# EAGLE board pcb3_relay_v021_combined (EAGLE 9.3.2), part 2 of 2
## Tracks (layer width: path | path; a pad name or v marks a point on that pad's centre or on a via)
+5V  (via drill 0.35)
  Top 0.61: 21.59,26.04 v21.59,19.43 21.59,10.03 21.08,9.53 IC1.10 | 21.59,26.04 v21.59,36.07 | IC2.16 19.68,33.66 v20.32,34.29 | IC1.16 19.68,17.14 v20.32,17.78 | IC2.10 21.59,26.04
  Top 1.016: C8.1 C30.+ 22.99,72.39 26.42,68.96 v26.42,36.07
  Bottom 0.61: v20.32,34.29 C2.1 | v20.32,17.78 C1.1 17.91,19.05 18.29,19.43 v21.59,19.43
  Bottom 1.016: C8.1 IC4.3 | C2.1 17.91,35.44 18.54,36.07 v21.59,36.07 v26.42,36.07
  other vias: 22.73,72.39
+12V  (via drill 0.35)
  Top 1.016: C15.+ C16.1 22.99,62.36 21.59,60.96 21.59,55.88 22.86,54.61 22.86,30.48 | v27.18,29.46 26.17,30.47 K1.1 22.86,30.48 | v37.34,29.46 36.33,30.47 K2.1 | v47.5,29.46 46.49,30.47 K3.1 | v57.66,29.46 56.65,30.47 K4.1 | v67.82,29.46 66.81,30.47 K5.1 | v77.98,29.46 76.97,30.47 K6.1 | v88.14,29.46 87.13,30.47 K7.1 | v98.3,29.46 97.29,30.47 K8.1 | v108.46,29.46 107.45,30.47 K9.1 | v118.62,29.46 117.61,30.47 K10.1 | v128.78,29.46 127.77,30.47 K11.1 | v138.94,29.46 137.93,30.47 K12.1 | v149.1,29.46 148.09,30.47 K13.1 | v159.26,29.46 158.25,30.47 K14.1 | v169.42,29.46 168.41,30.47 K28.1 | v37.34,10.41 36.33,11.42 K16.1 | K15.1 26.17,11.42 v27.18,10.41 27.18,16 22.86,20.32 22.86,30.48 | v47.5,10.41 46.49,11.42 K17.1 | v57.66,10.41 56.65,11.42 K18.1 | v67.82,10.41 66.81,11.42 K19.1 | v77.98,10.41 76.97,11.42 K20.1 | v88.14,10.41 87.13,11.42 K21.1 | v98.3,10.41 97.29,11.42 K22.1 | v108.46,10.41 107.45,11.42 K23.1 | v118.62,10.41 117.61,11.42 K24.1 | v128.78,10.41 127.77,11.42 K25.1 | v138.94,10.41 137.93,11.42 K26.1 | v149.1,10.41 148.09,11.42 K27.1 | v169.42,10.41 168.41,11.42 K29.1 | IC3.3 v17.78,62.23
  Bottom 1.016: IC4.1 22.86,67.31 24.13,66.04 C16.1 24,62.23 v17.78,62.23 | DS1.C 27.16,29.45 v27.18,29.46 32.89,29.46 33.27,29.08 35.56,29.08 35.94,29.46 v37.34,29.46 | v37.34,29.46 v47.5,29.46 | v47.5,29.46 v57.66,29.46 | v57.66,29.46 v67.82,29.46 | v67.82,29.46 v77.98,29.46 | v77.98,29.46 v88.14,29.46 | v88.14,29.46 v98.3,29.46 | v98.3,29.46 v108.46,29.46 | v108.46,29.46 v118.62,29.46 | v118.62,29.46 v128.78,29.46 | v128.78,29.46 v138.94,29.46 | v138.94,29.46 v149.1,29.46 | v149.1,29.46 v159.26,29.46 | v159.26,29.46 v169.42,29.46 169.4,29.45 DS28.C | DS2.C 37.34,27.96 v37.34,29.46 | DS3.C 47.48,29.45 v47.5,29.46 | DS4.C 57.64,29.45 v57.66,29.46 | DS5.C 67.8,29.45 v67.82,29.46 | DS6.C 77.96,29.45 v77.98,29.46 | DS7.C 88.12,29.45 v88.14,29.46 | DS14.C 159.24,29.45 v159.26,29.46 | DS13.C 149.08,29.45 v149.1,29.46 | DS12.C 138.92,29.45 v138.94,29.46 | DS11.C 128.76,29.45 v128.78,29.46 | DS10.C 118.6,29.45 v118.62,29.46 | DS9.C 108.44,29.45 v108.46,29.46 | DS8.C 98.28,29.45 v98.3,29.46 | v37.34,10.41 v27.18,10.41 27.16,10.4 DS15.C | DS16.C 37.34,8.91 v37.34,10.41 | v37.34,10.41 v47.5,10.41 | DS17.C 47.48,10.4 v47.5,10.41 | v47.5,10.41 v57.66,10.41 | DS18.C 57.66,8.91 v57.66,10.41 | v57.66,10.41 v67.82,10.41 | DS19.C 67.8,10.4 v67.82,10.41 | v67.82,10.41 v77.98,10.41 | DS20.C 77.96,10.4 v77.98,10.41 | v77.98,10.41 v88.14,10.41 | DS21.C 88.14,8.91 v88.14,10.41 | v88.14,10.41 v98.3,10.41 | DS22.C 98.28,10.4 v98.3,10.41 | v98.3,10.41 v108.46,10.41 | DS23.C 108.46,8.91 v108.46,10.41 | v108.46,10.41 v118.62,10.41 | DS24.C 118.6,10.4 v118.62,10.41 | v118.62,10.41 v128.78,10.41 | DS25.C 128.76,10.4 v128.78,10.41 | v128.78,10.41 v138.94,10.41 | DS26.C 138.94,8.91 v138.94,10.41
  Bottom 1.016: v138.94,10.41 v149.1,10.41 | DS27.C 149.08,10.4 v149.1,10.41 | v149.1,10.41 v169.42,10.41 169.42,8.91 DS29.C
  other vias: 24.13,62.36
+15V  (via drill 0.35)
  Top 0.61: IC38.4 158.75,68.45 C38P.1 | IC35.7 153.03,51.44 153.67,52.07 v154.94,52.07 | IC36.7 167,51.44 167.64,52.07 v170.18,52.07 | IC37.7 179.71,51.82 180.21,52.32 182.63,52.32 v182.88,52.07 | IC32.7 126.36,47.62 127,48.26 v128.27,48.26 129.54,49.53 v129.54,52.7 v129.54,58.42 128.27,59.69 v128.27,66.04 | IC31.7 36.2,64.14 36.83,64.77 v38.1,64.77 39.37,63.5 39.37,62.23 38.1,60.96 v38.1,45.72 | IC25.7 52.7,64.64 53.09,65.02 54.48,65.02 54.76,64.75 v54.76,64.64 | IC28.7 52.7,49.15 53.31,49.76 54.51,49.76 v54.68,49.59 v54.67,49.59 | R157.2 R135.2 | IC30.8 97.16,47.88 97.41,48.13 v99.06,48.13 v99.06,58.42 102.87,62.23 v102.87,67.18 101.22,67.18 100.97,66.93 IC27.8 | IC34.7 132.72,68.07 132.97,68.33 134.62,68.33 v134.62,68.2 | v176.53,65.41 E49.TP | IC33.7 122.56,69.09 122.94,69.47 124.84,69.47 v124.97,69.34
  Top 1.016: +15V.TP 5.08,45.72 C66.+ C60.1 | C14.1 C18.+ 16.76,45.72 17.78,46.74 IC3.1 C70.+
  Bottom 0.61: v154.94,52.07 C35P.1 154.94,48.9 | v170.18,52.07 170.56,51.69 C36P.1 170.56,48.9 | v182.88,52.07 C37P.1 182.88,49.53 182.25,48.9 170.56,48.9 | C32P.1 v128.27,48.26 132.08,48.26 132.87,49.05 152.72,49.05 152.88,48.9 154.94,48.9 | v38.1,64.77 C31P.1 C25P.1 54.76,63.52 v54.76,64.64 | v54.67,49.59 54.67,48.19 C28P.1 54.61,45.72 | C14.1 16.26,45.84 16.26,46.61 16.72,47.08 22.77,47.08 24.13,45.72 v38.1,45.72 54.61,45.72 | R157.2 85.26,45.72 84.24,44.7 83.4,44.7 82.38,45.72 54.61,45.72 | v99.06,48.13 C30P.1 | v102.87,67.18 C27P.1 | v134.62,68.2 C34P.1 134.62,65.41 | R135.2 87.63,58.42 v99.06,58.42 v129.54,58.42 | 170.56,48.9 154.94,48.9 | v176.53,65.41 160.02,65.41 | 160.02,65.41 134.62,65.41 | 134.62,65.41 128.91,65.41 v128.27,66.04 125.86,68.45 C33P.1 v124.97,69.34 | R198.1 161.29,76.45 161.8,76.96 176.02,76.96 176.53,77.47 E49.TP | C38P.1 160.02,67.18 160.02,65.41
  Bottom 1.016: C60.1 7.49,46.61 8.38,47.5 12.83,47.5 14.61,45.72 C14.1
  other vias: 159.89,67.31 7.49,45.72 16.38,45.72
-15V  (via drill 0.35)
  Top 0.61: IC31.4 33.66,69.47 33.4,69.72 31.88,69.72 31.75,69.6 C31N.2 v31.75,58.42 | IC25.4 50.16,69.6 49.78,69.98 48.51,69.98 48.26,69.72 C25N.2 v48.26,58.42 48.26,54.48 | IC28.4 50.16,54.48 49.91,54.74 48.51,54.74 48.26,54.48 | 48.26,54.48 C28N.2 | IC30.4 93.34,53.21 93.09,53.47 91.82,53.47 91.44,53.09 | 91.44,53.09 C30N.2 | IC27.4 97.16,72.26 96.9,72.52 v95.25,72.52 | IC32.4 123.83,52.96 123.57,53.21 122.17,53.21 121.92,52.96 C32N.2 v121.92,55.88 | IC33.4 120.02,73.28 119.76,73.53 118.36,73.53 118.11,73.28 C33N.2 v118.11,55.88 | IC34.4 130.18,73.28 129.92,73.53 128.52,73.53 128.27,73.28 C34N.2 | IC35.4 150.5,56.77 150.24,57.02 148.84,57.02 148.59,56.77 C35N.2 | IC36.4 164.47,56.77 164.21,57.02 162.94,57.02 162.56,56.64 | 162.56,56.64 C36N.2 | IC37.4 177.16,57.02 176.91,57.28 175.64,57.28 175.26,56.9 C37N.2 | v162.56,60.96 162.56,56.64 | v158.75,62.1 IC38.11 158.75,66.8 v158.5,67.06 | 91.44,53.09 v91.44,55.88 91.44,69.85 v92.71,71.12 | IC26.14 80.01,57.15 v81.28,55.88 81.28,52.07 80.01,50.8 IC29.14 | v7.62,57.15 7.46,57.3 C71.-
  Top 1.016: -15V.TP 5.08,68.58 C67.- v8.13,68.58 8.13,65.91 7.46,65.25 C71.-
  Bottom 0.61: C37N.2 175,55.75 162.82,55.75 C36N.2 162.56,57.15 162.05,57.66 149.1,57.66 148.59,57.15 C35N.2 122.05,56.01 v121.92,55.88 v118.11,55.88 v91.44,55.88 v81.28,55.88 80.16,57 R152.1 62.08,57.15 60.96,57.15 59.69,58.42 v48.26,58.42 v31.75,58.42 29.21,58.42 27.94,57.15 v7.62,57.15 | R195.1 164.95,60.96 v162.56,60.96 C38N.2 157.61,61.47 158.24,62.1 v158.75,62.1 | v158.5,67.06 158.39,67.16 R196.1 | v95.25,72.52 C27N.2 92.84,71.25 v92.71,71.12
  Bottom 1.016: v8.13,68.58 C61.2 | C33N.2 119.12,73.53 127.89,73.53 128.27,73.15 C34N.2
  other vias: 31.75,68.71 48.26,68.71 48.26,53.47 91.44,52.2 121.92,52.2 118.11,72.52 128.27,72.52 148.59,56.01 162.56,56.01 175.26,56.01
A01  (via drill 0.35)
  Top 0.305: v32.64,21.08 32.71,21.15 K1.5 | v42.8,21.08 42.87,21.15 K2.5 | v52.96,21.08 53.03,21.15 K3.5 | v63.12,21.08 63.19,21.15 K4.5 | v73.28,21.08 73.28,22.8 K5.5 | v83.44,21.08 83.51,21.15 K6.5 | v93.6,21.08 93.67,21.15 K7.5 | v103.76,21.08 103.76,22.8 K8.5 | v113.92,21.08 113.92,22.8 K9.5 | v124.08,21.08 124.08,22.8 K10.5 123.43,22.87 v122.17,24.13
  Bottom 0.305: RA1.1 25.25,21.49 25.65,21.08 v32.64,21.08 v42.8,21.08 v52.96,21.08 v63.12,21.08 v73.28,21.08 v83.44,21.08 v93.6,21.08 v103.76,21.08 v113.92,21.08 v124.08,21.08 | RB11.2 122.3,25.4 | 122.3,25.4 124.46,25.4 125.73,26.67 132.08,26.67 | 132.08,26.67 142.24,26.67 | 142.24,26.67 149.86,26.67 | 149.86,26.67 161.42,26.67 CAC4.2 | CAC3.1 149.73,26.54 149.86,26.67 | CAC2.2 142.37,26.54 142.24,26.67 | CAC1.2 132.21,26.54 132.08,26.67 | v122.17,24.13 122.17,25.27 122.3,25.4
A02  (via drill 0.35)
  Top 0.305: v25.65,1.65 25.71,1.71 K15.4 | v35.81,1.65 35.87,1.71 K16.4 | v45.97,1.65 46.03,1.71 K17.4 | v56.13,1.65 56.19,1.71 K18.4 | v66.29,1.65 66.35,1.71 K19.4 | v76.45,1.65 76.51,1.71 K20.4 | v86.61,1.65 86.67,1.71 K21.4 | v96.9,1.65 96.9,3.75 K22.4 | v106.93,1.65 106.99,1.71 K23.4 | v117.09,1.65 117.15,1.71 K24.4 | v127.25,1.65 127.31,1.71 K25.4 | v137.41,1.65 137.47,1.71 K26.4 v140.96,3.82 v140.97,3.81 | v147.57,1.65 147.63,1.71 K27.4 v151.12,3.82 v151.13,3.81 | v157.99,1.65 157.99,3.62 157.8,3.81 v156.21,3.81
  Bottom 0.305: v157.99,1.65 v147.58,1.65 v147.57,1.65 v137.41,1.65 v127.25,1.65 v117.09,1.65 v106.93,1.65 v96.9,1.65 v86.61,1.65 v76.45,1.65 v66.29,1.65 v56.13,1.65 v45.97,1.65 v35.82,1.65 v35.81,1.65 v25.65,1.65 23.75,1.65 22.86,2.54 RC1.1 | v140.97,3.81 CDF1.2 | CDF3.1 v156.21,3.81 | v151.13,3.81 CDF2.2
ACONT  (via drill 0.35)
  Top 0.305: IC27.1 100.97,72.26 v101.35,72.64 | C55.- v107.95,73.77 107.95,74.93 106.68,76.2 E23.TP | v87.63,73.66 87.63,77.47 CON1.8
  Bottom 0.305: v107.95,73.77 106.36,73.77 D16.2 104.73,72.64 v101.35,72.64 98.81,72.64 97.79,73.66 v87.63,73.66
AD_DIST  (via drill 0.35)
  Top 0.254: v116.84,78.74 v116.84,40.01
  Top 0.305: CON2.2 2.54,25.4 1.27,26.67 1.27,38.73 v2.54,40.01 | v179.07,46.99 177.67,45.59 v177.67,40.01
  Bottom 0.254: E42.TP v116.84,78.74
  Bottom 0.305: v177.67,40.01 v116.84,40.01 v2.54,40.01 | R1.2 v179.07,46.99 R193.1
E21  (via drill 0.35)
  Top 0.305: v43.18,46.99 E21.TP
  Bottom 0.305: R145.2 50.95,46.99 v43.18,46.99 | E21.TP 52.07,80.01 53.85,78.23 77.47,78.23 79.25,80.01 82.55,80.01 CON1.4
E29  (via drill 0.35)
  Top 0.305: E29.TP 30.48,39.37 29.21,38.1 v29.21,20.32 | v25.4,20.32 25.4,22.56 K1.4 | K2.4 35.56,22.56 v35.56,20.32 | v45.72,20.32 45.72,22.56 K3.4 | v55.88,20.32 55.88,22.56 K4.4 | v66.04,20.32 66.04,22.56 K5.4 | v76.2,20.32 76.2,22.56 K6.4 | v86.36,20.32 86.36,22.56 K7.4 | v96.52,20.32 96.52,22.56 K8.4 | v106.68,20.32 106.68,22.56 K9.4 | v116.84,20.32 116.84,22.56 K10.4 | R167.1 v35.56,78.74
  Bottom 0.305: v116.84,20.32 v106.68,20.32 v96.52,20.32 v86.36,20.32 v76.2,20.32 v66.04,20.32 v55.88,20.32 v45.72,20.32 v35.56,20.32 v29.21,20.32 v25.4,20.32 23.62,20.32 22.86,21.08 RB1.1 | E29.TP 31.75,78.74 v35.56,78.74 41.63,78.74 41.65,78.72 44.71,78.72 44.73,78.74 50.8,78.74 52.07,77.47 81.66,77.47 82.93,76.2 CON1.3
E31  (via drill 0.35)
  Top 0.305: IC38.2 v161.29,73.66 | v157.48,73.66 IC38.5 | E31.TP v113.03,76.2
  Bottom 0.305: v161.29,73.66 v157.48,73.66 143.51,73.66 140.97,76.2 v113.03,76.2 95.25,76.2 93.98,77.47 82.55,77.47 CON1.2
E32  (via drill 0.35)
  Top 0.305: C52.+ 69.85,71.63 73.66,75.44 v73.66,76.2 v73.66,80.01
  Bottom 0.305: E32.TP v73.66,80.01 | CON1.1 v73.66,76.2
E34  (via drill 0.35)
  Top 0.305: v129.67,20.95 v129.67,45.21
  Bottom 0.305: 150.11,20.95 157.35,20.95 | 157.35,20.95 166.62,20.95 | 166.62,20.95 170.81,20.95 171.32,21.46 171.32,22.84 R171.2 | CEG4.2 166.5,21.08 166.62,20.95 | CEG2.2 149.99,21.08 150.11,20.95 | CEG3.1 157.35,20.96 157.35,20.95 | 139.83,20.95 v129.67,20.95 129.69,20.98 RA11.2 | 139.83,20.95 150.11,20.95 | CEG1.2 139.83,20.96 139.83,20.95 | v129.67,45.21 126.36,45.21 125.73,45.85 R172.1
E35  (via drill 0.35)
  Top 0.305: K11.4 127.31,21.28 v128.27,20.32 | v137.16,20.32 137.47,20.63 K12.4 | v147.32,20.32 147.63,20.63 K13.4 | v157.48,20.32 157.79,20.63 K14.4 | v149.86,7.56 149.99,7.69 v149.99,20.32 | v130.81,20.32 130.81,27.43 130.69,27.55 v130.69,45.34 v130.68,45.34
  Bottom 0.305: 142.24,7.56 137.86,7.56 137.8,7.62 133.48,7.62 CBD1.2 | 142.24,7.56 v149.86,7.56 149.86,6.48 CBD3.1 | CBD2.2 142.24,6.48 142.24,7.56 | v128.27,20.32 v130.81,20.32 v137.16,20.32 v147.32,20.32 v149.99,20.32 v157.48,20.32 | R173.2 130.68,46.71 v130.68,45.34
E36  (via drill 0.35)
  Top 0.305: v32.64,2.29 32.71,2.36 K15.5 | v42.8,2.29 42.87,2.36 K16.5 | v52.96,2.29 53.03,2.36 K17.5 | v63.12,2.29 63.19,2.36 K18.5 | v73.28,2.29 73.35,2.36 K19.5 | v83.44,2.29 83.51,2.36 K20.5 | v93.6,2.29 93.67,2.36 K21.5 | v103.76,2.29 103.83,2.36 K22.5 | v113.92,2.29 113.99,2.36 K23.5 | v124.08,2.29 124.15,2.36 K24.5 | v134.24,2.29 134.31,2.36 K25.5 | v144.4,2.29 144.47,2.36 K26.5 | v154.56,2.29 154.63,2.36 K27.5 | v119.13,67.94 119.13,65.41 119.51,65.02 v119.51,2.29
  Bottom 0.305: RD1.1 25.25,2.56 25.53,2.29 v32.64,2.29 v42.8,2.29 v52.96,2.29 v63.12,2.29 v73.28,2.29 v83.44,2.29 v93.6,2.29 v103.76,2.29 v113.92,2.29 v119.51,2.29 v124.08,2.29 v134.24,2.29 v144.4,2.29 v154.56,2.29 | v119.13,67.94 119.61,68.43 R175.1 R174.2
E38  (via drill 0.35)
  Top 0.305: v125.73,6.35 125.73,13.46 125.48,13.71 125.48,35.82 125.73,36.08 125.73,64.52 v125.86,64.64
  Bottom 0.305: RC11.2 v125.73,6.35 | R207.1 v125.86,64.64
E40  (via drill 0.35)
  Top 0.305: v137.16,50.8 137.16,59.69 135.89,60.96 R180.1 v135.89,78.74 | IC34.6 v131.44,63.5 v131.45,63.5
  Bottom 0.305: R182.1 152.25,50.8 v137.16,50.8 | v135.89,78.74 E40.TP | R180.1 134.62,63.5 v131.45,63.5
E43
  Bottom 0.305: R200.2 E43.TP
E44
  Bottom 0.305: E44.TP 151.13,77.47 R201.2
E45
  Bottom 0.305: R202.2 E45.TP
E46  (via drill 0.35)
  Top 0.305: v166.37,76.18 166.37,77.47 E46.TP
  Bottom 0.305: R203.2 v166.37,76.18
FCONT  (via drill 0.35)
  Top 0.305: IC38.9 v156.21,62.99 | v160.02,62.99 IC38.12 | IC30.1 v97.16,53.72 | C59.- v104.14,53.72 107.95,57.53 v107.95,61.59 107.95,62.23 105.41,64.77 v105.41,75.05 | v100.33,74.93 E22.TP
  Bottom 0.305: v160.02,62.99 v156.21,62.99 154.43,62.99 153.67,62.23 138.43,62.23 137.16,60.96 120.65,60.96 120.02,61.59 v107.95,61.59 | v97.16,53.72 v104.14,53.72 109.81,53.72 D21.2 | v105.41,75.05 100.45,75.05 v100.33,74.93 92.71,74.93 91.44,76.2 CON1.7
GND  (via drill 0.35)
  Top 0.305: K28.3 169.37,25.07 v169.42,25.02 | IC34.3 v131.44,73.91
  Bottom 0.305: RD11.2 v132.08,3.81 | R199.1 v163.83,76.18 | C36P.2 v170.56,54.74
  pour Top (isolate 0.406): 0,82.55 189.23,82.55 189.23,0 0,0
  pour Bottom (isolate 0.305): 0,82.55 189.23,82.55 189.23,0 0,0
N$1  (via drill 0.35)
  Top 0.305: v70.87,66.02 70.87,65.02 72.39,63.5 IC26.8
  Bottom 0.305: v70.87,66.02 70.98,66.14 R130.1
N$2  (via drill 0.35)
  Top 0.305: R192.1 v184.15,45.72
  Bottom 0.305: v184.15,45.72 184.15,46.84 R193.2
N$3  (via drill 0.35)
  Top 0.305: IC37.3 v178.44,57.53
  Bottom 0.305: v178.44,57.53 180.09,57.53 180.34,57.28 R190.2
N$4  (via drill 0.35)
  Top 0.305: IC36.2 167,55.24 v167.64,54.61
  Bottom 0.305: v167.64,54.61 R186.1 R187.2 164.41,53.49 163.59,54.31 160.51,54.31 R185.1
N$5  (via drill 0.35)
  Top 0.305: v167,43.81 167,44.83 165.1,46.73 v165.1,52.07
  Bottom 0.305: D23.1 v167,43.81 | v165.1,52.07 R187.1
N$6  (via drill 0.35)
  Top 0.305: IC36.6 v165.74,46.99 | v162.56,43.81 v162.56,46.99
  Bottom 0.305: v165.74,46.99 D22.1 v162.56,46.99 | D23.2 v162.56,43.81
N$7  (via drill 0.35)
  Top 0.305: v172.72,49.68 v172.72,46.99 | v169.06,50.8 169.06,47.01 v169.04,46.99
  Bottom 0.305: R188.1 v172.72,49.68 | v172.72,46.99 v169.04,46.99 D22.2 | R186.2 167.79,50.8 v169.06,50.8
N$8  (via drill 0.35)
  Top 0.305: v172.72,54.61 v172.72,58.42 | v179.71,58.42 IC37.2 | C74.- v185.42,58.42
  Bottom 0.305: R188.2 v172.72,54.61 | R189.1 172.87,58.27 v172.72,58.42 177.8,58.42 | v185.42,58.42 v179.71,58.42 177.8,58.42 | R191.1 177.8,57.15 177.8,57.53 177.8,58.42
N$9  (via drill 0.35)
  Top 0.305: v177.86,52.13 178.44,51.55 IC37.6 178.44,48.9 180.34,46.99 180.34,43.18 | 180.34,43.18 R192.3 | 180.34,43.18 R192.2 | C74.+ v185.42,44.45
  Bottom 0.305: v177.86,52.13 177.8,52.18 R191.2 | v185.42,44.45 182.88,44.45 R192.2
N$10  (via drill 0.35)
  Top 0.305: C73.- 160.02,57.15 | 160.02,57.15 v160.02,58.44 | v158.75,56.87 159.03,57.15 160.02,57.15
  Bottom 0.305: v160.02,58.44 160.04,58.42 168.76,58.42 R189.2 | R185.2 159.38,56.24 v158.75,56.87
N$11  (via drill 0.35)
  Top 0.305: IC38.13 v161.29,63.12
  Bottom 0.305: R194.2 R195.2 163.98,63.65 163.45,63.12 v161.29,63.12
N$12  (via drill 0.35)
  Top 0.305: IC38.3 160.02,72.26 v160.15,72.39
  Bottom 0.305: v160.15,72.39 161.14,72.39 R198.2 R199.2
N$13  (via drill 0.35)
  Top 0.305: v156.21,71.12 IC38.6
  Bottom 0.305: R196.2 v156.21,71.12 154.79,71.12 R197.2
N$14  (via drill 0.35)
  Top 0.305: IC38.1 v162.56,73.66
  Bottom 0.305: R203.1 166.37,73.28 165.99,73.66 v162.56,73.66
N$15  (via drill 0.35)
  Top 0.305: v171.45,76.18 E47.TP
  Bottom 0.305: R204.2 v171.45,76.18
N$16  (via drill 0.35)
  Top 0.305: IC35.2 153.03,59.05 v152.4,59.69
  Bottom 0.305: R183.1 R184.2 v152.4,59.69
N$17  (via drill 0.35)
  Top 0.305: IC25.2 52.7,70.48 50.95,72.24 R127.1 v50.8,73.66
  Bottom 0.305: R125.1 v50.8,73.66
N$18  (via drill 0.35)
  Top 0.305: IC38.7 154.94,71.88 v155.19,72.14
  Bottom 0.305: v155.19,72.14 155.3,72.24 R202.1
N$19  (via drill 0.35)
  Top 0.305: v153.67,69.85 153.67,68.58 154.94,67.31 IC38.8
  Bottom 0.305: v153.67,69.85 152.4,69.85 151.13,71.12 R201.1
N$20  (via drill 0.35)
  Top 0.305: v25.65,26.04 25.71,25.98 K1.3
  Bottom 0.305: RB2.1 27.64,25.55 25.65,25.55 | 25.65,25.55 RB1.2 | v25.65,26.04 25.65,25.55
N$21
  Top 0.305: R179.2 136.04,58.9 133.35,61.59 R180.2
  Bottom 0.305: R180.3 R180.2
N$22
  Top 0.305: R127.2 R126.1 55.6,75.08 D12.1 D13.2
N$23  (via drill 0.35)
  Top 0.305: v35.31,26.04 35.31,25.65 35.87,25.09 K2.3
  Bottom 0.305: RB2.2 31.27,26.04 v35.31,26.04 37.31,26.04 RB3.1
N$24  (via drill 0.35)
  Top 0.305: D13.1 D12.2 | D12.2 55.6,72.24 R126.2 | IC25.6 51.44,65.41 v52.07,66.04 | C53.+ 58.31,65.07 v58.31,67.31 58.31,69.53 D12.2
  Bottom 0.305: v52.07,66.04 53.34,67.31 v58.31,67.31
N$25  (via drill 0.35)
  Top 0.305: v163.83,68.58 162.56,67.31 IC38.14 | v146.05,68.58 v146.05,71.12
  Bottom 0.305: v146.05,71.12 R200.1 | v163.83,68.58 v146.05,68.58
N$26  (via drill 0.35)
  Top 0.305: v45.47,26.16 45.47,25.63 K3.3
  Bottom 0.305: RB3.2 41.55,26.16 v45.47,26.16 47.35,26.16 RB4.1
N$27  (via drill 0.35)
  Top 0.305: v53.34,57 52.7,56.36 IC28.2 52.7,52.32 v52.07,51.69
  Bottom 0.305: R146.1 v53.34,57 54.33,57 D17.1 D18.2 | v52.07,51.69 R145.1
N$28  (via drill 0.35)
  Top 0.305: C56.- 58.61,53.34 v59.69,53.34
  Bottom 0.305: v59.69,53.34 58.57,52.22 | 58.57,52.22 R147.1 | R148.2 62.23,49.53 59.54,52.22 58.57,52.22
N$29  (via drill 0.35)
  Top 0.305: IC28.6 51.44,45.09 v52.07,44.45 | v58.42,44.45 C56.+ 58.42,49.53 56.52,51.44 v56.52,60.12
  Bottom 0.305: D18.1 v56.52,60.12 D17.2 52.35,60.12 R146.2 | v52.07,44.45 v58.42,44.45
N$30  (via drill 0.35)
  Top 0.305: IC26.3 v77.47,64.77
  Bottom 0.305: v77.47,64.77 77.32,64.62 R137.2
N$31  (via drill 0.35)
  Top 0.305: v81.28,69.34 81.28,67.42 81.39,67.31 81.39,66.79 81.28,66.68 v81.28,58.4 | IC26.10 v74.93,59.69
  Bottom 0.305: R129.1 v81.28,69.34 | v81.28,58.4 81.26,58.42 81.26,58.44 80.01,59.69 v74.93,59.69
N$32  (via drill 0.35)
  Top 0.305: K4.3 55.86,25.4 55.86,26.05 v55.75,26.16
  Bottom 0.305: RB4.2 51.71,26.16 v55.75,26.16 57.51,26.16 RB5.1
N$33  (via drill 0.35)
  Top 0.305: IC32.6 v125.09,44.45 v125.1,44.45 | v131.44,44.45 v131.44,50.93 v131.44,55.12 | IC32.2 v126.36,55.12
  Bottom 0.305: v125.1,44.45 v131.44,44.45 | v126.36,55.12 v131.44,55.12 | R173.1 130.56,50.04 v131.44,50.93
N$34  (via drill 0.35)
  Top 0.305: IC32.3 125.09,50.42 v124.33,49.66
  Bottom 0.305: v124.33,49.66 124.36,49.68 R172.2
N$35  (via drill 0.35)
  Top 0.305: IC29.2 v78.74,53.34
  Bottom 0.305: v78.74,53.34 78.74,52.22 R159.1
N$36  (via drill 0.35)
  Top 0.305: v82.55,59.69 82.55,58.42 R135.3
  Bottom 0.305: R134.1 v82.55,59.69
N$37  (via drill 0.35)
  Top 0.305: IC26.2 v78.74,63.5
  Bottom 0.305: v78.74,63.5 R137.1
N$38  (via drill 0.35)
  Top 0.305: IC26.5 v74.93,72.64 | v83.82,72.64 v83.82,66.04
  Bottom 0.305: v83.82,72.64 v74.93,72.64 | v83.82,66.04 78.89,66.04 R133.1
N$39  (via drill 0.35)
  Top 0.305: IC29.5 74.93,53.59 v74.42,53.09
  Bottom 0.305: v74.42,53.09 73.81,53.7 R155.1
N$40  (via drill 0.35)
  Top 0.305: IC29.8 72.39,50.8 v71.12,52.07
  Bottom 0.305: v71.12,52.07 R154.1
N$41  (via drill 0.35)
  Top 0.305: v76.2,74.91 IC26.4 | v67.31,74.93 v67.31,71.12
  Bottom 0.305: v67.31,71.12 R131.1 | v76.2,74.91 67.33,74.91 v67.31,74.93
N$42  (via drill 0.35)
  Top 0.305: IC26.1 80.76,66.95 v80.76,67.05
  Bottom 0.305: v80.76,67.05 77.47,67.05 77.06,67.46 R132.1
N$43  (via drill 0.35)
  Top 0.305: C52.- v69.85,73.91
  Bottom 0.305: R129.2 R128.1 78.64,73.91 v69.85,73.91
N$44  (via drill 0.35)
  Top 0.305: IC29.12 77.47,44.29 v78.74,43.02 | v85.09,52.07 v85.09,44.45
  Bottom 0.305: v78.74,43.02 78.9,43.18 80.14,43.18 C58.1 81.51,44.09 84.49,44.09 84.85,44.45 v85.09,44.45 | R156.2 84.94,52.22 v85.09,52.07 86.21,52.07 R160.2
N$45  (via drill 0.35)
  Top 0.305: v73.28,63.5 73.66,63.88 IC26.6 v73.66,68.58 | v85.09,64.77 v85.09,67.31
  Bottom 0.305: R139.1 72.26,62.21 C54.2 v73.28,63.5 | R136.1 v85.09,64.77 | v73.66,68.58 76.71,68.58 77.72,67.56 80.01,67.56 80.39,67.94 84.45,67.94 v85.09,67.31
N$46  (via drill 0.35)
  Top 0.305: IC26.12 77.47,62.02 v77.57,62.12
  Bottom 0.305: R138.2 87.63,63.5 86.36,62.23 82.55,62.23 | C54.1 76.39,62.17 77.28,62.17 77.33,62.12 v77.57,62.12 77.69,62.23 82.55,62.23 | R134.2 82.55,62.23
N$47  (via drill 0.35)
  Top 0.305: v96.65,68.58 97.16,68.07 IC27.5 97.16,59.84 v96.52,59.2
  Bottom 0.305: v96.65,68.58 R140.1 | v96.52,59.2 96.34,59.03 81.94,59.03 80.01,60.96 R139.2
N$48  (via drill 0.35)
  Top 0.305: IC27.6 98.42,64.77 v97.92,64.26
  Bottom 0.305: v97.92,64.26 97.79,64.14 R141.2 91.59,63.65 88.75,60.81 R138.1
N$49  (via drill 0.35)
  Top 0.305: IC29.10 v74.93,47.88
  Bottom 0.305: v74.93,47.88 74.93,48.41 R148.1
N$50  (via drill 0.35)
  Top 0.305: IC27.7 v99.69,60.81
  Bottom 0.305: D15.2 D14.1 102.39,60.02 R142.2 v99.69,60.81 R141.1
N$51
  Bottom 0.305: D15.1 D14.2 | D14.2 R143.2 | D14.2 101.83,63.42 R142.1
N$52  (via drill 0.35)
  Top 0.305: IC27.2 99.69,73.03 v100.33,73.66
  Bottom 0.305: R143.1 R144.2 108.38,69.16 D16.1 108.84,72.85 108.84,74.04 108.46,74.42 101.09,74.42 v100.33,73.66
N$53  (via drill 0.35)
  Top 0.305: v107.95,64.77 C55.+
  Bottom 0.305: R144.1 v107.95,64.77
N$54  (via drill 0.35)
  Top 0.305: v59.69,71.12 C53.- 60.77,67.31 v60.96,67.31
  Bottom 0.305: v59.69,71.12 R131.2 | R150.2 62.08,67.31 v60.96,67.31 59.84,67.31 R153.1
N$55  (via drill 0.35)
  Top 0.305: R135.1 88.9,58.42 87.63,59.69 v85.09,59.69
  Bottom 0.305: v85.09,59.69 R136.2
N$56  (via drill 0.35)
  Top 0.305: v60.96,58.42 v60.96,63.5 | IC29.4 76.2,57.76 v76.22,57.78
  Bottom 0.305: v60.96,58.42 63.5,58.42 64.14,57.78 v76.22,57.78 | v60.96,63.5 59.84,64.62 R153.2
N$57  (via drill 0.35)
  Top 0.305: IC29.3 v77.47,52.07
  Bottom 0.305: v77.47,52.07 R159.2
N$58
  Bottom 0.305: R157.3 R156.1
N$59  (via drill 0.35)
  Top 0.305: v88.9,50.8 R157.1
  Bottom 0.305: R158.2 82.7,50.8 v88.9,50.8
N$60  (via drill 0.35)
  Top 0.305: IC29.6 73.66,52.96 73.03,52.33 73.03,47.76 73.03,47.75 v73.03,47.12
  Bottom 0.305: R158.1 C58.2 81.26,47.14 R161.1 78.72,47.12 v73.03,47.12
N$61  (via drill 0.35)
  Top 0.305: v92.71,43.18 93.34,43.81 IC30.5 93.34,49.01 v92.82,49.53
  Bottom 0.305: v92.71,43.18 80.79,43.18 79.99,42.39 78.48,42.39 78.11,42.76 78.11,43.28 78.74,43.91 R161.2 | v92.82,49.53 R162.1
N$62  (via drill 0.35)
  Top 0.305: IC30.6 94.61,45.96 v94.49,45.83 | v90.04,49.4 v90.04,44.45
  Bottom 0.305: v94.49,45.83 91.93,45.83 91.29,45.19 R163.2 v90.04,44.45 | R160.1 90.02,49.38 v90.04,49.4
N$63
  Bottom 0.305: R165.1 101.6,44.45 102.87,45.72 D19.1 D20.2 106.96,46.84 R164.2
N$64  (via drill 0.35)
  Top 0.305: IC30.2 95.89,53.98 v96.52,54.61 | v107.95,54.61 v107.95,49.96 | v111.76,49.66 111.76,53.59 v112.14,53.98
  Bottom 0.305: D19.2 D20.1 v107.95,49.96 110.21,49.96 R164.1 111.78,49.68 | v96.52,54.61 v107.95,54.61 | R166.2 111.78,49.68 | 111.78,49.68 v111.76,49.66 | v112.14,53.98 D21.1
N$65  (via drill 0.35)
  Top 0.305: IC31.6 34.92,66.67 34.29,67.31 v34.29,77.47 | v45.72,77.47 C72.- | R170.1 v40.64,77.47
  Bottom 0.305: v34.29,77.47 v40.64,77.47 v45.72,77.47
N$66  (via drill 0.35)
  Top 0.305: v104.14,44.45 C59.+
  Bottom 0.305: R166.1 113.03,45.72 111.76,44.45 v104.14,44.45
N$67  (via drill 0.35)
  Top 0.305: IC29.1 80.01,55.96 v79.76,56.21
  Bottom 0.305: v79.76,56.21 67.9,56.21 67.46,55.78 R2.2
N$68  (via drill 0.35)
  Top 0.305: v64.64,63.37 v64.64,55.97
  Bottom 0.305: v64.64,63.37 64.64,64.49 R149.2 R132.2 | R2.1 64.62,55.95 v64.64,55.97
N$69  (via drill 0.35)
  Top 0.305: v67.31,69.85 C57.- | v63.5,59.69 v63.5,66.04
  Bottom 0.305: R149.1 64.92,67.46 | 64.92,67.46 v67.31,69.85 | R151.2 v63.5,59.69 63.35,59.84 R152.2 | 64.92,67.46 v63.5,66.04 62.23,64.77 R150.1
N$70  (via drill 0.35)
  Top 0.305: IC30.7 95.89,45.09 v95.25,44.45
  Bottom 0.305: R163.1 v95.25,44.45 R165.2
N$71
  Top 0.305: IC31.3 34.92,70.48 35.56,71.12 R167.2
N$72  (via drill 0.35)
  Top 0.305: R169.2 v40.64,40.64 | K28.4 166.74,22.87 166.45,23.16 166.45,34.24 167.13,34.92 v167.13,40.64
  Bottom 0.305: v40.64,40.64 165.87,40.64 v167.13,40.64
N$73
  Top 0.305: IC31.2 36.2,69.85 37.47,71.12 40.64,71.12 | R169.1 40.64,71.12 | 40.64,71.12 R170.2
N$74  (via drill 0.35)
  Top 0.305: v158.37,14.22 v158.37,9.14
  Bottom 0.305: D2.1 158.32,14.18 | 158.32,14.18 v158.37,14.22 | v158.37,9.14 158.62,8.89 RS31.1 | RS27.2 155.28,14.18 158.32,14.18 | D1.1 158.32,14.18
N$75  (via drill 0.35)
  Top 0.305: v120.65,69.85 121.28,70.48 IC33.3
  Bottom 0.305: R175.2 v120.65,69.85
N$76  (via drill 0.35)
  Top 0.305: v121.28,63.25 IC33.6 121.28,69.22 122.56,70.48 IC33.2
  Bottom 0.305: R176.1 122.3,62.23 v121.28,63.25 121.89,63.86 R207.2
N$79  (via drill 0.35)
  Top 0.305: v169.16,5.97 169.11,6.02 K29.3 166.7,6.02 166.37,6.35 166.37,10.54 165.74,11.17 v165.74,20.32 | v161.29,46.99 161.29,29.98 161.24,29.93 161.24,27.6 161.29,27.55 v161.29,20.32 | v133.35,60.33 134.62,59.05 v134.62,46.99 | v129.54,60.33 v129.54,62.23
  Bottom 0.305: R177.1 169.7,6.5 v169.16,5.97 | v165.74,20.32 v161.29,20.32 | v134.62,46.99 v161.29,46.99 | v133.35,60.33 v129.54,60.33 | v129.54,62.23 R176.2
N$80  (via drill 0.35)
  Top 0.305: K29.4 169.03,3.82 v169.16,3.68 170.31,4.83 170.31,44.7 v169.29,45.72 | IC34.2 132.72,70.23 132.08,69.6 132.08,55.88 | v132.08,45.72 132.08,55.88 | R179.1 132.08,55.88
  Bottom 0.305: v169.16,3.68 169.19,3.66 R177.2 | v169.29,45.72 v132.08,45.72
N$81  (via drill 0.35)
  Top 0.305: v152.4,54.61 151.76,55.24 IC35.3
  Bottom 0.305: R182.2 v152.4,54.61
N$84  (via drill 0.35)
  Top 0.305: v152.4,48.26 151.76,48.9 IC35.6 151.76,52.7 151.13,53.34 151.13,63.5 v151.26,63.63 | v160.02,48.11 C73.+
  Bottom 0.305: v152.4,48.26 159.87,48.26 v160.02,48.11 | R184.1 151.28,63.65 v151.26,63.63
N$85  (via drill 0.35)
  Top 0.305: v65.91,26.16 65.91,25.51 K5.3
  Bottom 0.305: RB5.2 61.87,26.16 v65.91,26.16 67.67,26.16 RB6.1
N$86  (via drill 0.35)
  Top 0.305: K6.3 76.18,25.4 76.18,25.93 v75.95,26.16
  Bottom 0.305: RB6.2 72.03,26.16 v75.95,26.16 77.83,26.16 RB7.1
N$87  (via drill 0.35)
  Top 0.305: v86.11,26.16 86.11,25.63 K7.3
  Bottom 0.305: RB7.2 82.19,26.16 v86.11,26.16 87.99,26.16 RB8.1
N$88  (via drill 0.35)
  Top 0.305: K8.3 96.5,25.4 96.5,26.05 v96.39,26.16
  Bottom 0.305: RB8.2 92.35,26.16 v96.39,26.16 98.15,26.16 RB9.1
N$89  (via drill 0.35)
  Top 0.305: v106.55,26.16 106.55,25.51 K9.3
  Bottom 0.305: RB9.2 102.51,26.16 v106.55,26.16 108.31,26.16 RB10.1
N$90  (via drill 0.35)
  Top 0.305: v116.59,26.16 116.59,25.63 K10.3
  Bottom 0.305: RB10.2 112.67,26.16 v116.59,26.16 118.47,26.16 RB11.1
N$91  (via drill 0.35)
  Top 0.305: v33.27,24 32.71,24.57 K1.6
  Bottom 0.305: RA1.2 29.23,24 v33.27,24 34.27,24 RA2.1
N$92  (via drill 0.35)
  Top 0.305: K2.6 42.87,25.09 43.43,24.53 v43.43,24
  Bottom 0.305: RA2.2 39.4,24 v43.43,24 44.42,24 RA3.1
N$93  (via drill 0.35)
  Top 0.305: K3.6 53.59,24.51 v53.59,24
  Bottom 0.305: RA3.2 49.55,24 v53.59,24 54.59,24 RA4.1
N$94  (via drill 0.35)
  Top 0.305: K4.6 63.5,24.76 v63.5,24
  Bottom 0.305: RA4.2 59.72,24 v63.5,24 64.75,24 RA5.1
N$95  (via drill 0.35)
  Top 0.305: v73.66,24.13 73.66,25.4 73.35,25.09 K5.6
  Bottom 0.305: RA5.2 70,24.13 v73.66,24.13 74.78,24.13 RA6.1
N$96  (via drill 0.35)
  Top 0.305: v83.82,24.13 83.82,25.4 83.51,25.09 K6.6
  Bottom 0.305: RA6.2 80.16,24.13 v83.82,24.13 84.94,24.13 RA7.1
N$97  (via drill 0.35)
  Top 0.305: v93.98,24.13 93.98,25.4 93.67,25.09 K7.6
  Bottom 0.305: RA7.2 90.32,24.13 v93.98,24.13 95.1,24.13 RA8.1
N$98  (via drill 0.35)
  Top 0.305: v104.14,24.13 104.14,25.4 103.83,25.09 K8.6
  Bottom 0.305: RA8.2 100.48,24.13 v104.14,24.13 105.26,24.13 RA9.1
N$99  (via drill 0.35)
  Top 0.305: K9.6 114.68,24.38 v114.68,24
  Bottom 0.305: RA9.2 110.52,24 v114.68,24 115.55,24 RA10.1
N$100  (via drill 0.35)
  Top 0.305: K10.6 123.83,24.75 v123.83,23.96
  Bottom 0.305: RA11.1 125.74,23.96 v123.83,23.96 123.41,23.96 122.3,22.86 RA10.2
N$101  (via drill 0.35)
  Top 0.305: v29.84,34.16 30.14,34.46 QS1.1
  Bottom 0.305: RS1.1 30.35,34.67 v29.84,34.16
N$102  (via drill 0.35)
  Top 0.508: QS1.3 31.75,30.6 31.62,30.47
  Top 1.016: v30.1,27.94 30.1,29.46 31.11,30.48 31.12,30.47 31.62,30.47 K1.8
  Bottom 1.016: DS1.A v30.1,27.94
N$103  (via drill 0.35)
  Top 0.305: v40.01,34.16 40.3,34.46 QS2.1
  Bottom 0.305: RS2.1 40.51,34.67 v40.01,34.16
N$104  (via drill 0.35)
  Top 0.508: QS2.3 41.91,30.47
  Top 1.016: v40.13,27.94 40.13,29.59 41.01,30.47 41.91,30.47 K2.8
  Bottom 1.016: DS2.A v40.13,27.94
N$105  (via drill 0.35)
  Top 0.305: v50.16,34.16 50.46,34.46 QS3.1
  Bottom 0.305: RS3.1 50.67,34.67 v50.16,34.16
N$106  (via drill 0.35)
  Top 0.508: QS3.3 52.07,30.47
  Top 1.016: v50.16,27.94 50.16,29.84 50.79,30.47 52.07,30.47 K3.8
  Bottom 1.016: DS3.A v50.16,27.94
N$107  (via drill 0.35)
  Top 0.305: v60.33,34.16 60.62,34.46 QS4.1
  Bottom 0.305: RS4.1 60.83,34.67 v60.33,34.16
N$108  (via drill 0.35)
  Top 0.508: QS4.3 62.23,30.6 62.1,30.47
  Top 1.016: v60.33,27.94 60.33,29.59 61.2,30.47 62.1,30.47 K4.8
  Bottom 1.016: DS4.A v60.33,27.94
N$109  (via drill 0.35)
  Top 0.305: QS5.1 71.14,34.16 v70.48,34.16
  Bottom 0.305: RS5.1 70.48,35.05 v70.48,34.16
N$110  (via drill 0.35)
  Top 0.508: QS5.3 72.39,30.6 72.26,30.47
  Top 1.016: v70.74,27.81 70.74,29.84 71.36,30.47 72.26,30.47 K5.8
  Bottom 1.016: DS5.A 71.77,27.81 v70.74,27.81
N$111  (via drill 0.35)
  Top 0.305: v80.52,34.16 80.81,34.46 QS6.1
  Bottom 0.305: RS6.1 81.15,34.8 v80.52,34.16
N$112  (via drill 0.35)
  Top 0.508: QS6.3 82.55,30.47
  Top 1.016: v80.64,27.81 80.64,29.46 81.65,30.47 82.55,30.47 K6.8
  Bottom 1.016: DS6.A 81.93,27.81 v80.64,27.81
N$113  (via drill 0.35)
  Top 0.305: v90.81,34.16 91.1,34.46 QS7.1
  Bottom 0.305: RS7.1 91.31,34.67 v90.81,34.16
N$114  (via drill 0.35)
  Top 0.508: QS7.3 92.71,30.47
  Top 1.016: v91.06,27.94 91.06,29.59 91.94,30.47 92.71,30.47 K7.8
  Bottom 1.016: DS7.A v91.06,27.94
N$115  (via drill 0.35)
  Top 0.305: v100.97,34.16 101.26,34.46 QS8.1
  Bottom 0.305: RS8.1 101.47,34.67 v100.97,34.16
N$116  (via drill 0.35)
  Top 0.508: QS8.3 102.87,30.6 102.74,30.47
  Top 1.016: v101.09,27.81 101.09,29.59 101.97,30.47 102.74,30.47 K8.8
  Bottom 1.016: DS8.A 102.25,27.81 v101.09,27.81
N$117  (via drill 0.35)
  Top 0.305: v111.12,34.16 111.42,34.46 QS9.1
  Bottom 0.305: RS9.1 111.63,34.67 v111.12,34.16
N$118  (via drill 0.35)
  Top 0.508: QS9.3 113.03,30.47
  Top 1.016: v111.25,27.81 111.25,29.72 112,30.47 113.03,30.47 K9.8
  Bottom 1.016: DS9.A 112.41,27.81 v111.25,27.81
N$119  (via drill 0.35)
  Top 0.305: v121.16,34.04 121.58,34.46 QS10.1
  Bottom 0.305: RS10.1 121.79,34.67 v121.16,34.04
N$120  (via drill 0.35)
  Top 0.508: QS10.3 123.19,30.6 123.32,30.47
  Top 1.016: v121.41,27.94 121.41,29.21 122.67,30.47 123.32,30.47 K10.8
  Bottom 1.016: DS10.A v121.41,27.94
N$121  (via drill 0.35)
  Top 0.305: K11.3 127.31,25.85 v127.25,25.91
  Bottom 0.305: v127.25,25.91 128.9,25.91 CAC1.1
N$122  (via drill 0.35)
  Top 0.305: K12.3 137.47,25.98 v137.41,26.04
  Bottom 0.305: v137.41,26.04 138.94,26.04 CAC2.1
N$123  (via drill 0.35)
  Top 0.305: K13.3 147.96,25.4 v151.13,25.4
  Bottom 0.305: v151.13,25.4 CAC3.2
N$124  (via drill 0.35)
  Top 0.305: v131.32,34.16 131.62,34.46 QS11.1
  Bottom 0.305: RS11.1 131.95,34.8 v131.32,34.16
N$125  (via drill 0.35)
  Top 0.508: QS11.3 133.35,30.47
  Top 1.016: v131.57,27.81 131.57,29.59 132.45,30.47 133.35,30.47 K11.8
  Bottom 1.016: DS11.A 132.73,27.81 v131.57,27.81
N$126  (via drill 0.35)
  Top 0.305: v141.6,34.16 141.9,34.46 QS12.1
  Bottom 0.305: RS12.1 142.11,34.67 v141.6,34.16
N$127  (via drill 0.35)
  Top 0.508: QS12.3 143.51,30.47
  Top 1.016: v141.86,27.94 141.86,29.59 142.74,30.47 143.51,30.47 K12.8
  Bottom 1.016: DS12.A v141.86,27.94
N$128  (via drill 0.35)
  Top 0.305: v151.64,34.16 151.94,34.46 QS13.1
  Bottom 0.305: RS13.1 152.27,34.8 v151.64,34.16
N$129  (via drill 0.35)
  Top 0.508: QS13.3 153.67,30.6 153.54,30.47
  Top 1.016: v151.89,27.94 151.89,29.46 152.9,30.47 153.54,30.47 K13.8
  Bottom 1.016: DS13.A v151.89,27.94
N$130  (via drill 0.35)
  Top 0.305: v161.93,34.16 162.22,34.46 QS14.1
  Bottom 0.305: RS14.1 162.43,34.67 v161.93,34.16
N$131  (via drill 0.35)
  Top 0.508: QS14.3 163.83,30.6 163.7,30.47
  Top 1.016: v162.05,27.94 162.05,29.59 162.93,30.47 163.7,30.47 K14.8
  Bottom 1.016: DS14.A v162.05,27.94
N$132  (via drill 0.35)
  Top 0.305: QS16.1 39.5,13.95 v39.5,12.57
  Bottom 0.305: v39.5,12.57 39.5,12.96 RS16.1
N$133  (via drill 0.35)
  Top 0.508: QS16.3 41.91,11.55 42.04,11.42
  Top 1.016: v40.13,8.89 40.13,10.41 41.14,11.42 42.04,11.42 K16.8
  Bottom 1.016: DS16.A v40.13,8.89
N$134  (via drill 0.35)
  Top 0.305: QS17.1 49.53,13.82 v49.53,12.7
  Bottom 0.305: RS17.1 49.53,12.83 v49.53,12.7
N$135  (via drill 0.35)
  Top 0.508: QS17.3 52.07,11.55 52.2,11.42
  Top 1.016: v50.29,8.89 50.29,10.41 51.3,11.42 52.2,11.42 K17.8
  Bottom 1.016: DS17.A v50.29,8.89
N$136  (via drill 0.35)
  Top 0.305: QS18.1 59.69,13.82 v59.69,12.7
  Bottom 0.305: v59.69,12.7 59.69,12.83 RS18.1
N$137  (via drill 0.35)
  Top 0.508: QS18.3 62.23,11.42
  Top 1.016: v60.58,8.89 60.58,10.54 61.46,11.42 62.23,11.42 K18.8
  Bottom 1.016: DS18.A v60.58,8.89
N$138  (via drill 0.35)
  Top 0.305: QS23.1 110.49,13.82 v110.49,12.7
  Bottom 0.305: RS23.1 110.49,12.83 v110.49,12.7
N$139  (via drill 0.35)
  Top 0.508: QS23.3 113.03,11.42
  Top 1.016: v111.38,8.76 111.38,10.67 112.13,11.42 113.03,11.42 K23.8
  Bottom 1.016: DS23.A 112.41,8.76 v111.38,8.76
N$140  (via drill 0.35)
  Top 0.305: v69.85,12.7 71.44,14.29 QS19.1
  Bottom 0.305: RS19.1 70.99,13.84 v69.85,12.7
N$141  (via drill 0.35)
  Top 0.508: QS19.3 72.39,11.42
  Top 1.016: v70.74,8.89 70.74,10.54 71.62,11.42 72.39,11.42 K19.8
  Bottom 1.016: DS19.A v70.74,8.89
N$142  (via drill 0.35)
  Top 0.305: QS20.1 81.6,14.29 v80.01,12.7
  Bottom 0.305: v80.01,12.7 81.15,13.84 RS20.1
N$143  (via drill 0.35)
  Top 0.508: QS20.3 82.55,11.55 82.68,11.42
  Top 1.016: v80.9,8.89 80.9,10.67 81.65,11.42 82.68,11.42 K20.8
  Bottom 1.016: DS20.A v80.9,8.89
N$144  (via drill 0.35)
  Top 0.305: QS21.1 90.17,13.82 v90.17,12.7
  Bottom 0.305: RS21.1 90.17,12.83 v90.17,12.7
N$145  (via drill 0.35)
  Top 0.508: QS21.3 92.71,11.42
  Top 1.016: v91.06,8.89 91.06,10.54 91.94,11.42 92.71,11.42 K21.8
  Bottom 1.016: DS21.A v91.06,8.89
N$146  (via drill 0.35)
  Top 0.305: QS22.1 100.33,13.82 v100.33,12.7
  Bottom 0.305: v100.33,12.7 100.33,12.83 RS22.1
N$147  (via drill 0.35)
  Top 0.508: QS22.3 102.87,11.55 103,11.42
  Top 1.016: v101.09,8.89 101.09,10.67 101.84,11.42 103,11.42 K22.8
  Bottom 1.016: DS22.A v101.09,8.89
N$148  (via drill 0.35)
  Top 0.305: v29.21,12.7 30.8,14.29 QS15.1
  Bottom 0.305: RS15.1 29.21,12.83 v29.21,12.7
N$149  (via drill 0.35)
  Top 0.508: QS15.3 31.75,11.42
  Top 1.016: v30.1,8.89 30.1,10.54 30.98,11.42 31.75,11.42 K15.8
  Bottom 1.016: DS15.A v30.1,8.89
N$151  (via drill 0.35)
  Top 0.305: IC2.14 v20.32,31.11 | v15.24,31.11 15.24,8.76 15.75,8.26 IC1.9
  Bottom 0.305: v20.32,31.11 v15.24,31.11
N$152  (via drill 0.35)
  Top 0.305: v134.37,24 134.37,25.01 K11.6
  Bottom 0.305: CEG1.1 135.89,24 v134.37,24
N$153  (via drill 0.35)
  Top 0.305: v144.53,24 144.53,25.01 K12.6
  Bottom 0.305: CEG2.1 146.05,24 v144.53,24
N$154  (via drill 0.35)
  Top 0.305: K13.6 155.32,24.38 v155.32,24
  Bottom 0.305: v155.32,24 156.36,24 156.42,24.07 159.7,24.07 160.27,23.5 160.15,23.37 CEG3.2
N$155  (via drill 0.35)
  Top 0.305: K14.3 158.24,25.52 v158.24,26.04
  Bottom 0.305: v158.24,26.04 159.25,26.04 CAC4.1
N$156  (via drill 0.35)
  Top 0.305: v165.1,24.13 165.1,24.76 K14.6
  Bottom 0.305: CEG4.1 164.97,24.13 v165.1,24.13
N$157  (via drill 0.35)
  Top 0.305: v25.78,6.99 25.71,6.91 K15.3
  Bottom 0.305: RC1.2 25.78,6.5 | 25.78,6.5 27.64,6.5 RC2.1 | v25.78,6.99 25.78,6.5
N$158  (via drill 0.35)
  Top 0.305: v34.29,6.35 35.54,6.35 K16.3
  Bottom 0.305: RC2.2 v34.29,6.35 RC3.1
N$159  (via drill 0.35)
  Top 0.305: v44.45,6.35 45.7,6.35 K17.3
  Bottom 0.305: RC3.2 v44.45,6.35 RC4.1
N$160  (via drill 0.35)
  Top 0.305: v54.61,6.35 55.86,6.35 K18.3
  Bottom 0.305: RC4.2 v54.61,6.35 RC5.1
N$161  (via drill 0.35)
  Top 0.305: v64.77,6.35 66.02,6.35 K19.3
  Bottom 0.305: RC5.2 v64.77,6.35 RC6.1
N$162  (via drill 0.35)
  Top 0.305: v74.93,6.35 75.26,6.02 K20.3
  Bottom 0.305: RC6.2 v74.93,6.35 RC7.1
N$163  (via drill 0.35)
  Top 0.305: v85.09,6.35 85.42,6.02 K21.3
  Bottom 0.305: RC7.2 v85.09,6.35 RC8.1
N$164  (via drill 0.35)
  Top 0.305: v95.25,6.35 96.5,6.35 K22.3
  Bottom 0.305: RC8.2 v95.25,6.35 RC9.1
N$165  (via drill 0.35)
  Top 0.305: v105.41,6.35 106.66,6.35 K23.3
  Bottom 0.305: RC9.2 v105.41,6.35 RC10.1
N$166  (via drill 0.35)
  Top 0.305: v115.57,6.35 116.82,6.35 K24.3
  Bottom 0.305: RC10.2 v115.57,6.35 RC11.1
N$167  (via drill 0.35)
  Top 0.305: v34.29,3.81 34.29,4.44 K15.6
  Bottom 0.305: RD1.2 v34.29,3.81 RD2.1
N$168  (via drill 0.35)
  Top 0.305: v44.45,3.81 44.45,5.08 43.18,6.35 42.87,6.04 K16.6
  Bottom 0.305: RD2.2 v44.45,3.81 RD3.1
N$169  (via drill 0.35)
  Top 0.305: v54.61,3.81 54.61,5.08 53.34,6.35 53.34,6.33 K17.6
  Bottom 0.305: RD3.2 v54.61,3.81 RD4.1
N$170  (via drill 0.35)
  Top 0.305: v64.77,3.81 64.77,5.08 63.5,6.35 63.19,6.04 K18.6
  Bottom 0.305: RD4.2 v64.77,3.81 RD5.1
N$171  (via drill 0.35)
  Top 0.305: v74.93,3.81 74.93,5.08 73.66,6.35 73.35,6.04 K19.6
  Bottom 0.305: RD5.2 v74.93,3.81 RD6.1
N$172  (via drill 0.35)
  Top 0.305: v85.09,3.81 85.09,5.08 83.82,6.35 83.51,6.04 K20.6
  Bottom 0.305: RD6.2 v85.09,3.81 RD7.1
N$173  (via drill 0.35)
  Top 0.305: v95.25,3.81 95.25,5.08 93.98,6.35 93.67,6.04 K21.6
  Bottom 0.305: RD7.2 v95.25,3.81 RD8.1
N$174  (via drill 0.35)
  Top 0.305: v105.41,3.81 105.41,5.08 104.14,6.35 103.83,6.04 K22.6
  Bottom 0.305: RD8.2 v105.41,3.81 RD9.1
N$175  (via drill 0.35)
  Top 0.305: v115.57,3.81 115.57,5.08 114.3,6.35 113.99,6.04 K23.6
  Bottom 0.305: RD9.2 v115.57,3.81 RD10.1
N$176  (via drill 0.35)
  Top 0.305: v125.73,3.81 125.73,5.08 124.46,6.35 124.15,6.04 K24.6
  Bottom 0.305: RD10.2 v125.73,3.81 RD11.1
N$177  (via drill 0.35)
  Top 0.305: v127.25,7.11 127.25,6.08 K25.3
  Bottom 0.305: CBD1.1 128.02,6.35 v127.25,7.11
N$178  (via drill 0.35)
  Top 0.305: v137.54,6.99 137.47,6.91 K26.3
  Bottom 0.305: CBD2.1 138.18,6.35 v137.54,6.99
N$179  (via drill 0.35)
  Top 0.305: K27.3 147.65,6.02 v148.59,5.08
  Bottom 0.305: v148.59,5.08 148.66,5.14 150.66,5.14 151.86,6.35 CBD3.2
N$180  (via drill 0.35)
  Top 0.305: v135.76,5.97 135.71,6.02 K25.6
  Bottom 0.305: CDF1.1 135.76,5.08 v135.76,5.97
N$181  (via drill 0.35)
  Top 0.305: K26.6 146.18,4.31 v146.18,3.68
  Bottom 0.305: v146.18,3.68 147.06,3.68 CDF2.1
N$182  (via drill 0.35)
  Top 0.305: K27.6 155.57,5.08 v155.96,5.08
  Bottom 0.305: v155.96,5.08 160.02,5.08 160.15,4.95 CDF3.2
N$183  (via drill 0.35)
  Top 0.305: QS27.1 151.13,13.82 v151.13,12.7
  Bottom 0.305: RS27.1 151.13,12.83 v151.13,12.7
N$184  (via drill 0.35)
  Top 0.508: QS27.3 153.67,11.42
  Top 1.016: v152.02,8.76 152.02,10.79 152.64,11.42 153.67,11.42 K27.8
  Bottom 1.016: DS27.A 153.05,8.76 v152.02,8.76
N$185  (via drill 0.35)
  Top 0.305: QS24.1 122.24,14.29 v120.65,12.7
  Bottom 0.305: v120.65,12.7 121.79,13.84 RS24.1
N$186  (via drill 0.35)
  Top 0.508: QS24.3 123.19,11.55 123.32,11.42
  Top 1.016: v121.54,8.89 121.54,10.92 122.04,11.42 123.32,11.42 K24.8
  Bottom 1.016: DS24.A v121.54,8.89
N$187  (via drill 0.35)
  Top 0.305: v130.81,12.7 132.4,14.29 QS25.1
  Bottom 0.305: RS25.1 131.95,13.84 v130.81,12.7
N$188  (via drill 0.35)
  Top 0.508: QS25.3 133.35,11.42
  Top 1.016: v131.57,8.89 131.57,10.79 132.2,11.42 133.35,11.42 K25.8
  Bottom 1.016: DS25.A v131.57,8.89
N$189  (via drill 0.35)
  Top 0.305: QS26.1 142.56,14.29 v140.97,12.7
  Bottom 0.305: v140.97,12.7 142.11,13.84 RS26.1
N$190  (via drill 0.35)
  Top 0.508: QS26.3 143.51,11.42
  Top 1.016: v141.86,8.89 141.86,10.54 142.74,11.42 143.51,11.42 K26.8
  Bottom 1.016: DS26.A v141.86,8.89
N$193  (via drill 0.35)
  Top 0.305: v171.96,34.16 172.25,34.46 QS28.1
  Bottom 0.305: RS28.1 172.59,34.8 v171.96,34.16
N$194  (via drill 0.35)
  Top 0.508: QS28.3 173.99,30.6 173.86,30.47
  Top 1.016: v172.21,27.94 172.21,29.84 172.84,30.47 173.86,30.47 K28.8
  Bottom 1.016: DS28.A v172.21,27.94
N$195  (via drill 0.35)
  Top 0.305: v171.45,12.7 173.04,14.29 QS29.1
  Bottom 0.305: RS29.1 172.59,13.84 v171.45,12.7
N$196  (via drill 0.35)
  Top 0.508: QS29.3 173.99,11.55 174.12,11.42
  Top 1.016: v172.21,8.76 172.21,10.79 172.84,11.42 174.12,11.42 K29.8
  Bottom 1.016: DS29.A 173.37,8.76 v172.21,8.76
R01  (via drill 0.35)
  Top 0.305: v34.29,13.97 v34.29,30.1 v34.29,35.56 | IC2.7 v10.16,26.04
  Bottom 0.305: RS1.2 v34.29,35.56 | v34.29,13.97 RS15.2 | v10.16,26.04 20.45,26.04 21.07,26.66 23.1,26.66 26.72,30.28 34.11,30.28 v34.29,30.1
R02  (via drill 0.35)
  Top 0.305: v44.45,35.56 v44.45,30.61 v44.45,13.97 | IC2.6 12.08,27.21 v10.16,27.21
  Bottom 0.305: RS2.2 v44.45,35.56 | v44.45,13.97 RS16.2 | v10.16,27.21 17.97,27.21 18.51,26.67 20.33,26.67 20.77,27.11 22.91,27.11 26.53,30.73 44.22,30.73 44.27,30.79 v44.45,30.61
R03  (via drill 0.35)
  Top 0.305: v54.61,35.56 v54.61,31.07 v54.61,13.97 | IC2.5 10.26,28.57 v10.16,28.48
  Bottom 0.305: RS3.2 v54.61,35.56 | v54.61,13.97 RS17.2 | v10.16,28.48 19.27,28.48 19.81,27.94 23.03,27.94 26.34,31.24 54.44,31.24 v54.61,31.07
R04  (via drill 0.35)
  Top 0.305: v64.77,35.56 v64.77,31.47 v64.77,13.97 | IC2.4 v10.16,29.84
  Bottom 0.305: RS4.2 v64.77,35.56 | v64.77,13.97 RS18.2 | v64.77,31.47 64.54,31.7 26.15,31.7 24.29,29.84 v10.16,29.84
R05  (via drill 0.35)
  Top 0.305: v74.93,35.56 v74.93,31.88 v74.93,13.97 | IC2.3 v10.16,31.11
  Bottom 0.305: RS5.2 v74.93,35.56 | v74.93,13.97 RS19.2 | v10.16,31.11 11.18,31.11 11.81,30.48 24.28,30.48 25.96,32.16 73.64,32.16 73.66,32.13 74.68,32.13 v74.93,31.88
R06  (via drill 0.35)
  Top 0.305: v85.09,35.56 v85.09,32.38 v85.09,13.97 | IC2.2 v10.16,32.38
  Bottom 0.305: RS6.2 v85.09,35.56 | v85.09,13.97 RS20.2 | v10.16,32.38 10.29,32.26 25.41,32.26 25.77,32.61 84.86,32.61 v85.09,32.38
R07  (via drill 0.35)
  Top 0.305: v95.25,35.56 v95.25,33.78 v95.25,13.97 | IC2.1 v10.41,33.66
  Bottom 0.305: RS7.2 v95.25,35.56 | v95.25,13.97 RS21.2 | v10.41,33.66 13.61,33.66 14.18,33.09 20,33.09 20.45,33.53 95,33.53 v95.25,33.78
R08  (via drill 0.35)
  Top 0.305: v105.41,35.56 v105.41,33.07 v105.41,13.97 | IC2.15 20.19,32.38 v20.7,32.89
  Bottom 0.305: RS8.2 v105.41,35.56 | v105.41,13.97 RS22.2 | v20.7,32.89 25.4,32.89 25.58,33.07 v105.41,33.07
R09  (via drill 0.35)
  Top 0.305: v115.57,35.56 v115.57,16.28 v115.57,13.97 | IC1.7 v10.16,9.53
  Bottom 0.305: RS9.2 v115.57,35.56 | v115.57,13.97 RS23.2 | v10.16,9.53 20.46,9.53 27.39,16.46 115.39,16.46 v115.57,16.28
R10  (via drill 0.35)
  Top 0.305: IC1.6 v10.17,10.79 v10.16,10.8 | v126.11,13.97 v126.11,16.74 126.11,22.14 126.11,31.2 v126.11,35.56
  Bottom 0.305: RS24.2 v126.11,13.97 | v126.11,35.56 RS10.2 | v10.16,10.8 18.38,10.8 19.02,10.16 20.45,10.16 27.2,16.92 125.93,16.92 v126.11,16.74
R11  (via drill 0.35)
  Top 0.305: v135.89,35.56 v135.89,17.2 v135.89,13.97 | IC1.5 v10.16,12.06 v10.16,12.07
  Bottom 0.305: RS11.2 v135.89,35.56 | v135.89,13.97 RS25.2 | v135.89,17.2 135.72,17.37 26.52,17.37 20.58,11.43 19.05,11.43 18.41,12.07 v10.16,12.07
R12  (via drill 0.35)
  Top 0.305: v146.05,35.56 v146.05,17.65 v146.05,13.97 | IC1.4 v10.16,13.34
  Bottom 0.305: RS12.2 v146.05,35.56 | v146.05,13.97 RS26.2 | v10.16,13.34 20.99,13.34 25.49,17.83 145.87,17.83 v146.05,17.65
R13  (via drill 0.35)
  Top 0.305: v156.21,35.56 v156.21,18.14 | IC1.3 v10.16,14.61 | v163.83,18.14 v163.83,15.88
  Bottom 0.305: v156.21,35.56 RS13.2 | v10.16,14.61 19.17,14.61 19.8,13.97 20.98,13.97 25.3,18.29 156.06,18.29 v156.21,18.14 v163.83,18.14 | v163.83,15.88 D1.2
R14  (via drill 0.35)
  Top 0.305: v166.37,12.7 v166.37,19.05 166.37,22.23 166,22.6 166,35.19 v166.37,35.56 | IC1.2 v10.16,15.88
  Bottom 0.305: RS14.2 v166.37,35.56 | v10.16,15.88 10.79,16.51 22.23,16.51 24.95,19.23 166.19,19.23 v166.37,19.05 | v166.37,12.7 D2.2
R15  (via drill 0.35)
  Top 0.305: IC1.1 10.79,17.14 10.16,17.78 v10.16,20.32 | v176.53,19.68 v176.53,35.56
  Bottom 0.305: v10.16,20.32 21.59,20.32 22.23,19.69 v176.53,19.69 v176.53,19.68 | v176.53,35.56 RS28.2
R16  (via drill 0.35)
  Top 0.305: IC1.15 v20.07,15.88 | v176.53,18.88 v176.53,13.97
  Bottom 0.305: v20.07,15.88 22.24,15.88 25.14,18.77 165.75,18.77 166.11,18.42 176.07,18.42 v176.53,18.88 | v176.53,13.97 RS29.2
SDIN  (via drill 0.35)
  Top 0.305: v8.25,31.75 v8.25,15.88 | v20.07,14.61 IC1.14
  Bottom 0.305: CON2.8 5.08,31.75 v8.25,31.75 | v8.25,15.88 8.89,15.24 19.43,15.24 v20.07,14.61
SHCP  (via drill 0.35)
  Top 0.305: IC2.11 v20.07,27.3 | v7.62,12.06 v7.62,28.32 7.62,32.89 7.49,33.02 CON2.7 | v20.07,10.79 IC1.11
  Bottom 0.305: v7.62,28.32 8.09,27.85 18.64,27.85 19.18,27.3 v20.07,27.3 | v20.07,10.79 19.04,10.79 18.4,11.44 10.42,11.44 10.16,11.44 8.25,11.44 v7.62,12.06
SIG  (via drill 0.35)
  Top 0.305: v45.72,69.85 C72.+
  Bottom 0.305: R125.2 45.72,72.54 v45.72,69.85
STCP  (via drill 0.35)
  Top 0.305: IC2.12 v20.07,28.57 | CON2.5 5.08,29.21 v5.08,12.7 | v20.07,12.06 IC1.12
  Bottom 0.305: v5.08,12.7 19.43,12.7 v20.07,12.06 | v20.07,28.57 19.53,29.11 7.72,29.11 CON2.5

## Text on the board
tDocu: QREF | POWER SUPPLY | IREF | DIST. / IN | HIGH LOW / FREQ. LEDS | HIGH LOW / LEVEL LEDS | PWR / LED | +15V | FCONT | ACONT | DIST. ADC | DIST. OUT | GND | D | AGC | THD Analyzer B. Cordell / PCB 3, v0.21, 2022-05 / PCB by Emile | DIST. CAL. | AMPLITUDE AND / FREQUENCY DETECTORS | METER CIRCUIT / AND LEDS | FILTERS | METER / LEVEL / CAL. | RELAYS + DIGITAL
bDocu: THD-Analyzer / B. Cordell / PCB3, v0.21 by Emile / Bottom-Layer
